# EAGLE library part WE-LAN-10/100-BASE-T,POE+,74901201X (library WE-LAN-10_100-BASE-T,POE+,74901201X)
LAN-Transformer WE-LAN 10/100 Base Tx - Compliant with IEEE 802.3 standards - SMD -- Ethernet -- Power over Ethernet -- 1 Gigabit Ethernet -- Compliant with most IC's for ethernet applications like Intel, AMD, Globespan and Realtek -- Hub, Router, Switch
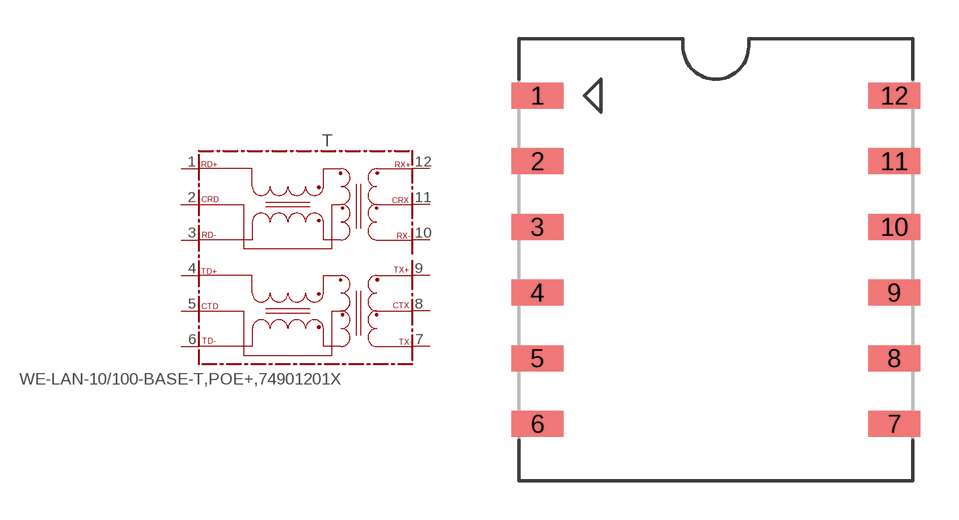
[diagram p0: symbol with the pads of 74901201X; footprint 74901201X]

Designator prefix T

## WE-LAN-10/100-BASE-T,POE+,74901201X(749012011) (MPN: 749012011; OC_FARNELL: 1636365; OC_NEWARK: 08P2941; PACKAGE: 10/100/Base T PoE+; SUPPLIER: Wuerth Elektronik)  [74901201X]
1  RD+
2  CRD
3  RD-
4  TD+
5  CTD
6  TD-
7  TX-
8  CTX
9  TX+
10  RX-
11  CRX
12  RX+

## WE-LAN-10/100-BASE-T,POE+,74901201X(749012013)  [74901201X]
Pads as for 74901201X

## Footprint 74901201X (pad centres in mm)
MAX Height = 8.4mm
smd 2 x 1: 1 -6.9,6.35; 2 -6.9,3.81; 3 -6.9,1.27; 4 -6.9,-1.27; 5 -6.9,-3.81; 6 -6.9,-6.35; 7 6.9,-6.35; 8 6.9,-3.81; 9 6.9,-1.27; 10 6.9,1.27; 11 6.9,3.81; 12 6.9,6.35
